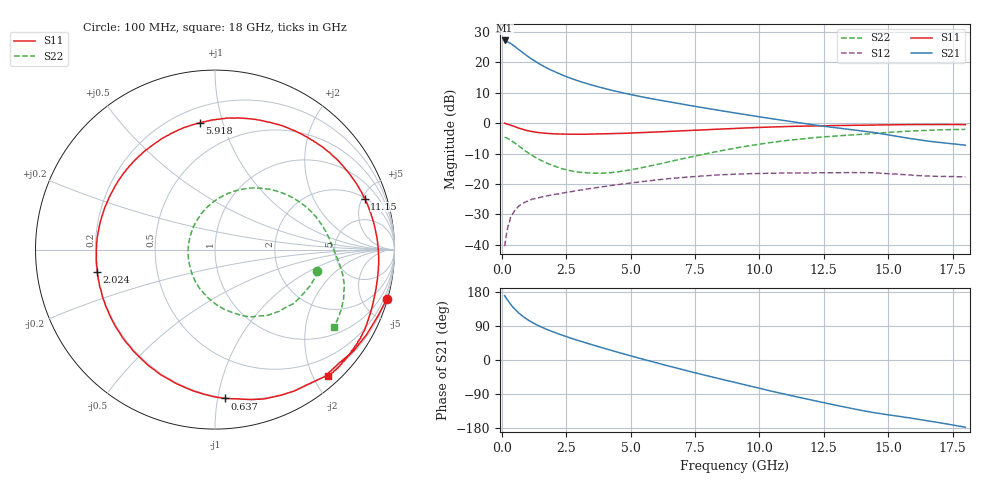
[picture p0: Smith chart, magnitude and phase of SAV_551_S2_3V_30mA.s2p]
! Data provided by Modelithics, Inc.  Tampa, Florida USA, June 2008
!Model SAV-551+
!VAR V_out= 3
!VAR I_out= 30
!VAR V_in= 0.3772
!VAR I_in= 0.8792
!BEGIN ACDATA
# GHZ S MA R 50
! Scattering Parameters
!% F n11x n11y n21x n21y n12x n12y n22x n22y
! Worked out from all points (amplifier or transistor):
!   401 points, 100 MHz to 18 GHz, reference 50 ohm
!   highest |S21| = 27.2 dB at 100 MHz (marker M1)
!   |S21| within 3 dB of that: start of sweep to 653 MHz
!   unconditionally stable (mu >= 1): 4.114 GHz to 10.51 GHz
!   at 3.054 GHz: K = 0.88, MSG = 17.9 dB, |S12| = -22.1 dB
!   at 9.05 GHz: K = 1.05, MAG = 8.8 dB, |S12| = -16.8 dB
!   at 18 GHz: K = 0.89, MSG = 5.2 dB, |S12| = -17.7 dB
!   lowest NFmin = 0.08 dB at 500 MHz
!   S11 on the Smith chart (normalised r, x): 100 MHz: 0.10, -7.06; 637 MHz: 0.20, -1.05; 2.024 GHz: 0.20, -0.09; 5.918 GHz: 0.29, +0.84; 11.15 GHz: 2.06, +5.25; 18 GHz: 0.17, -2.23
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0.1  0.9962 -16.1  22.99 169.9  0.00942 80.2  0.5819 -11.8
0.1895  0.9684 -29.2  21.99 160.6  0.01653 75.0  0.5678 -20.4
0.279  0.9376 -42.2  21.07 151.9  0.0222 68.3  0.5419 -29.9
0.3685  0.9125 -55.2  20.07 144.0  0.02937 62.1  0.5095 -39.1
0.50275  0.8757 -71.9  18.27 133.8  0.03698 53.3  0.4692 -51.2
0.637  0.8315 -86.1  16.48 124.8  0.04251 48.5  0.4283 -61.2
0.77125  0.7971 -98.5  14.87 117.2  0.04685 43.7  0.3855 -69.8
0.9055  0.7668 -109.6  13.46 110.4  0.05037 40.1  0.3499 -77.7
1.174  0.7257 -128.7  11.2 99.1  0.05607 33.6  0.2933 -91.9
1.532  0.6909 -148.3  9.044 86.8  0.06072 28.5  0.2413 -107.8
2.02425  0.668 -169.1  7.084 73.1  0.06666 23.9  0.1973 -127.0
2.47175  0.6591 175.7  5.889 62.2  0.07235 20.3  0.1721 -143.1
3.09825  0.6556 157.6  4.751 48.5  0.07971 16.3  0.1539 -165.0
4.396  0.673 126.8  3.372 22.4  0.09524 6.0  0.1561 153.2
5.9175  0.712 96.9  2.476 -6.0  0.1149 -8.2  0.2042 114.9
6.0965  0.7176 93.7  2.399 -9.1  0.1167 -10.0  0.2128 111.4
7.439  0.762 71.3  1.904 -32.7  0.1317 -24.1  0.284 86.6
9.05  0.8167 47.4  1.47 -59.5  0.1441 -41.9  0.3872 61.7
11.15325  0.8813 18.8  1.069 -92.8  0.1513 -66.2  0.5223 33.1
12.04825  0.8987 7.9  0.9433 -106.0  0.1515 -76.3  0.5721 22.4
15.0465  0.9363 -23.2  0.6373 -145.0  0.1469 -106.7  0.7049 -7.9
18  0.9446 -48.2  0.4335 -177.3  0.1305 -131.4  0.7896 -33.1
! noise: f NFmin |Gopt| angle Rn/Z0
0.5  0.076  0.3342  41.65  0.056
0.7  0.107  0.3406  50.02  0.051
0.9  0.138  0.3471  58.35  0.046
1  0.154  0.3503  62.5  0.044
1.9  0.294  0.3798  99.47  0.033
2.4  0.371  0.3964  119.7  0.032
3  0.465  0.4166  143.7  0.036
3.9  0.604  0.4473  179.1  0.054
5  0.775  0.4855  -138.6  0.092
6  0.93  0.521  -101.1  0.144
